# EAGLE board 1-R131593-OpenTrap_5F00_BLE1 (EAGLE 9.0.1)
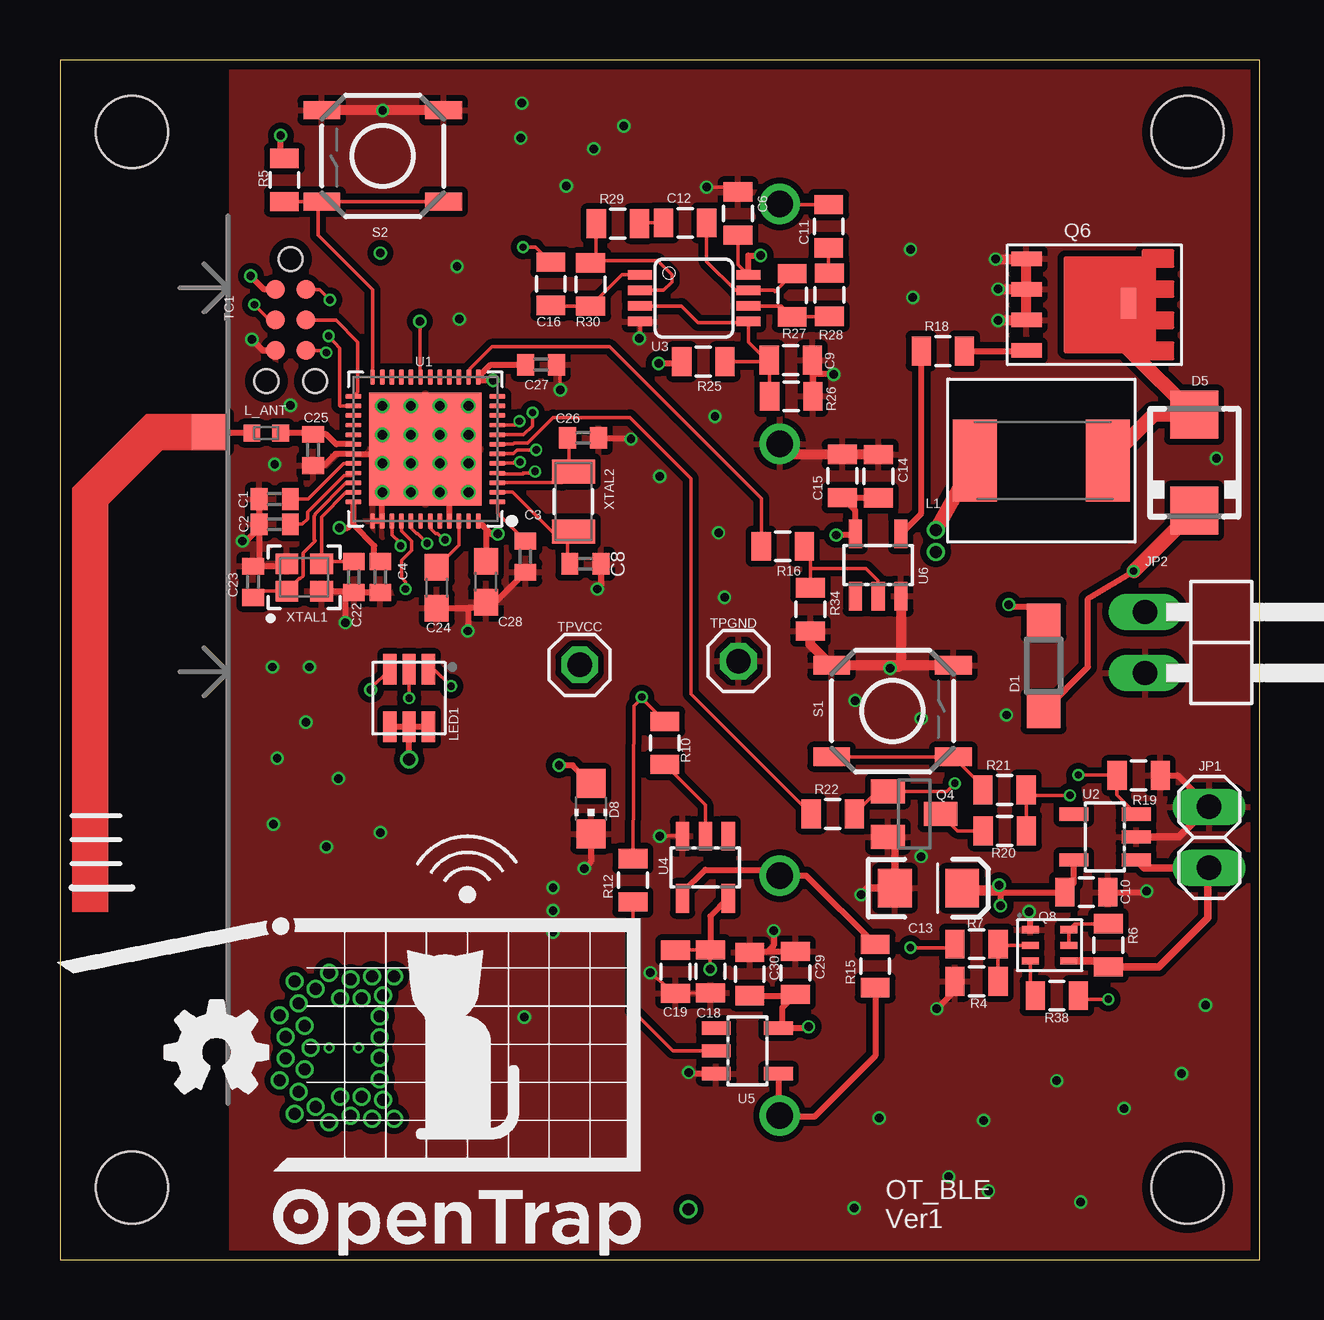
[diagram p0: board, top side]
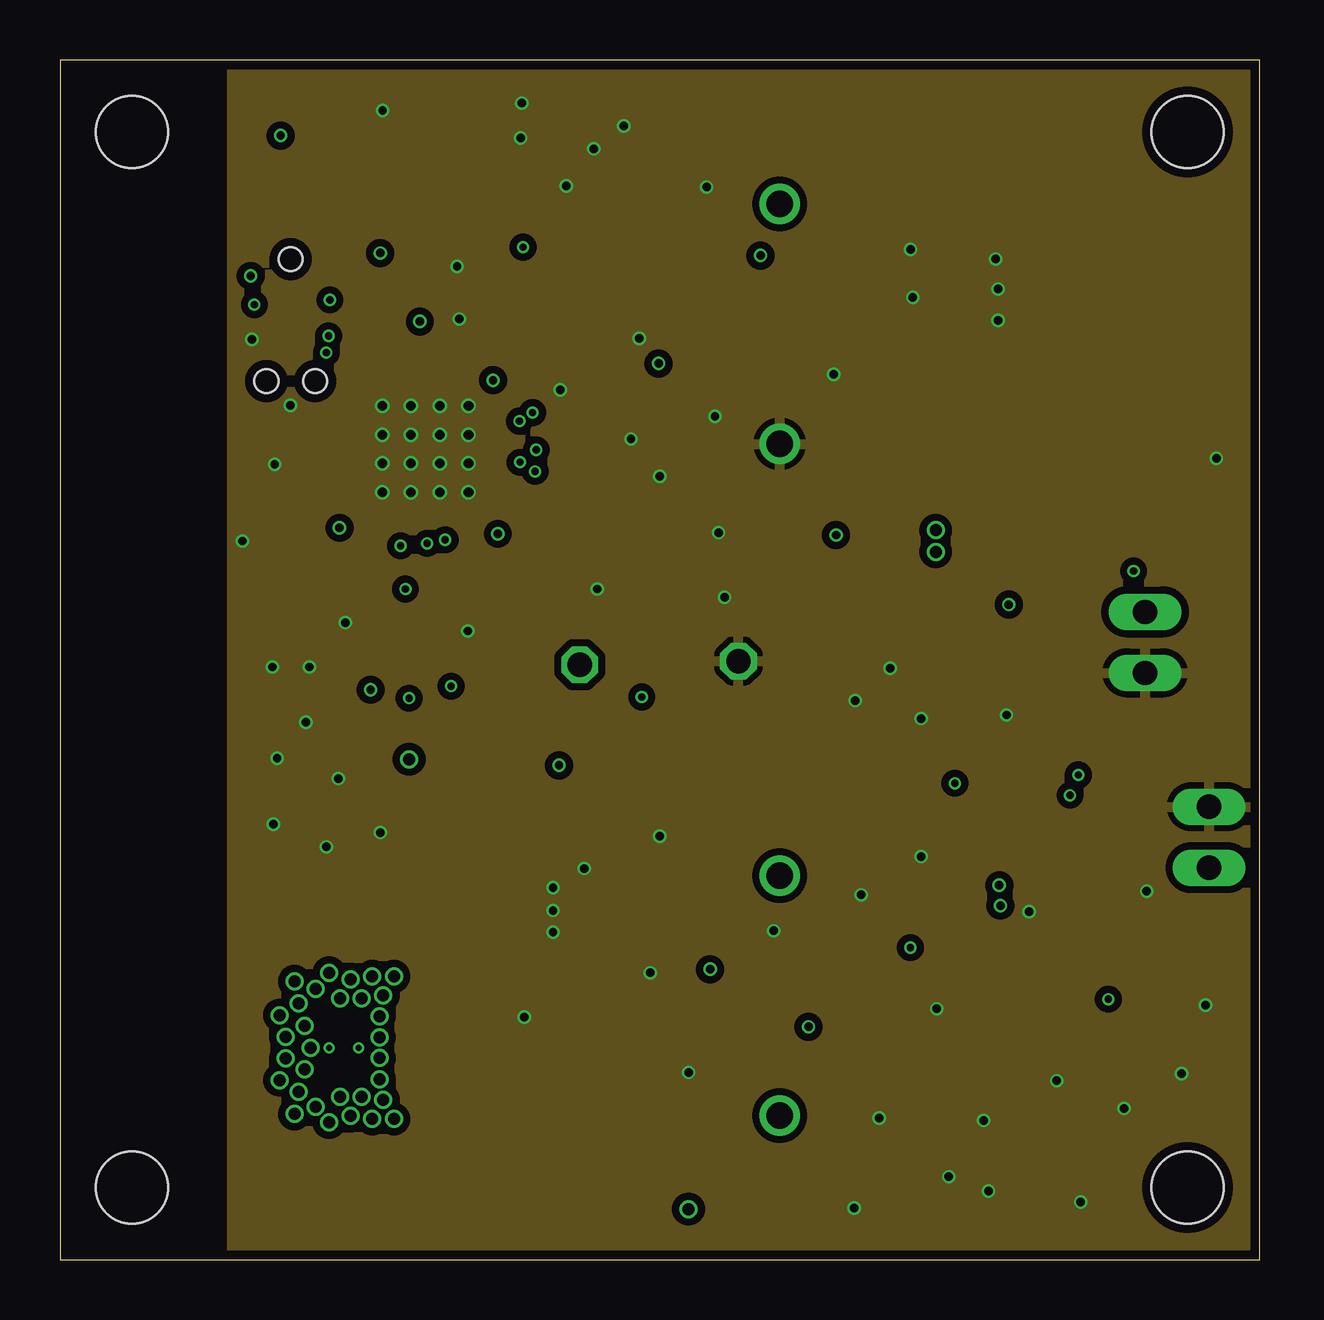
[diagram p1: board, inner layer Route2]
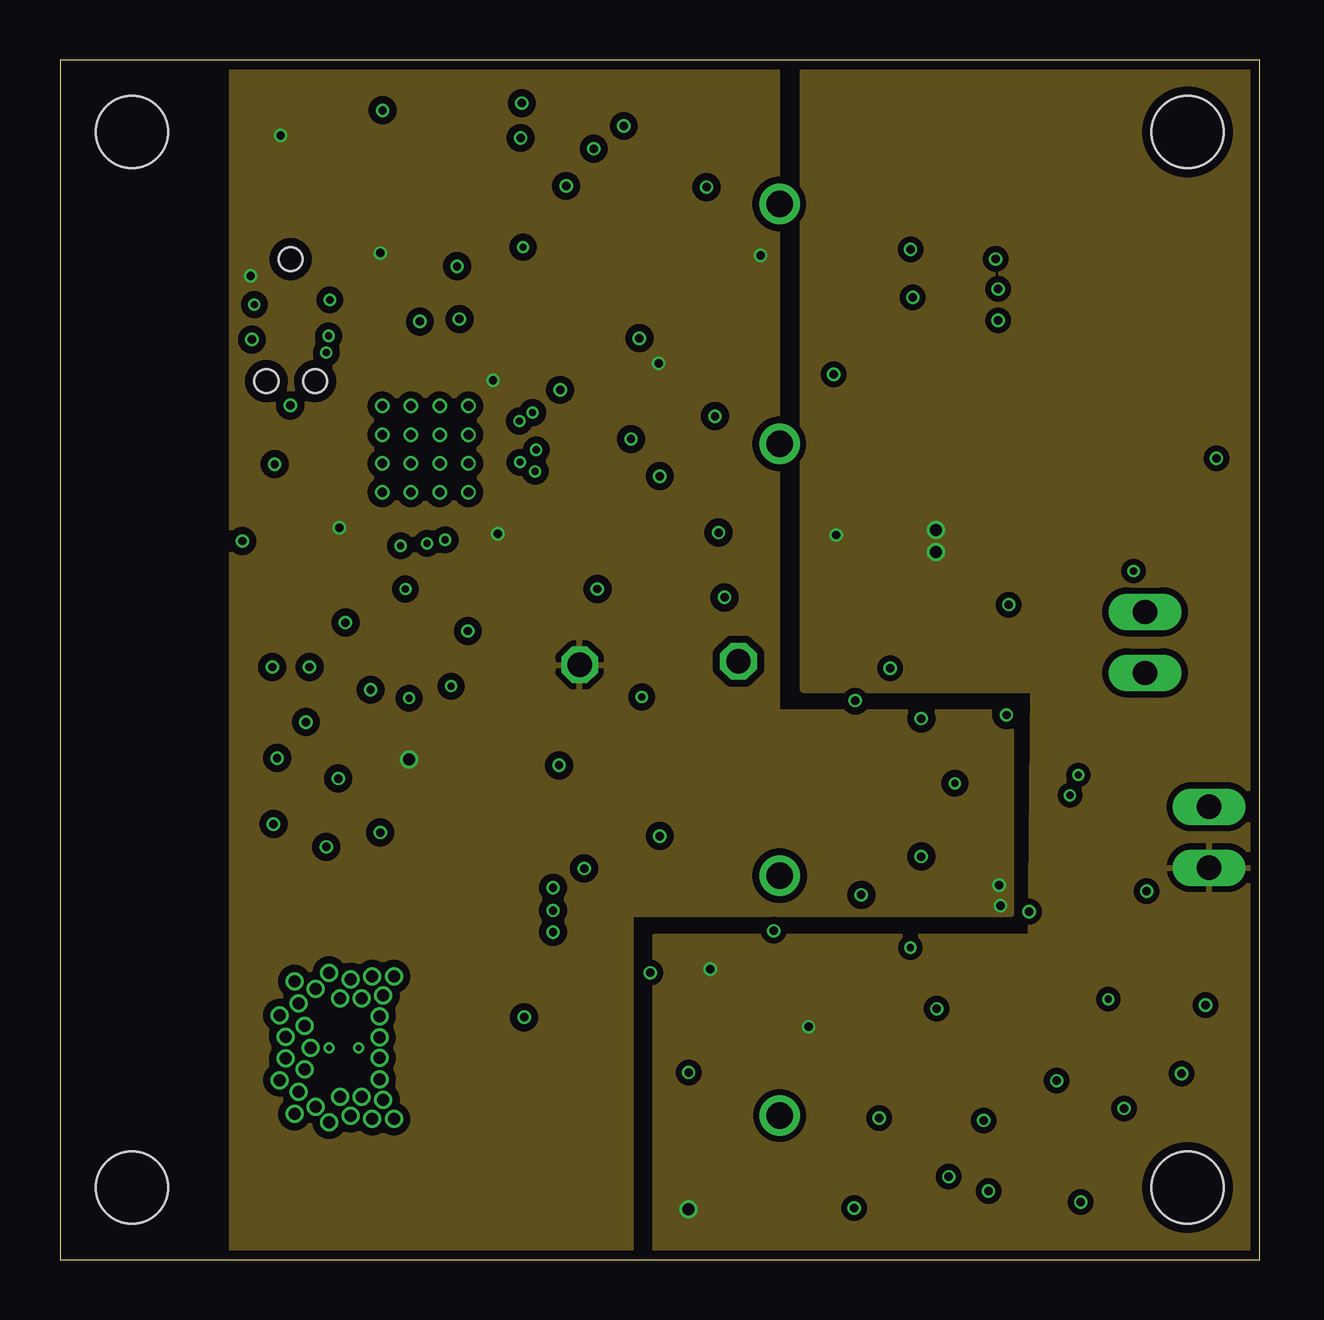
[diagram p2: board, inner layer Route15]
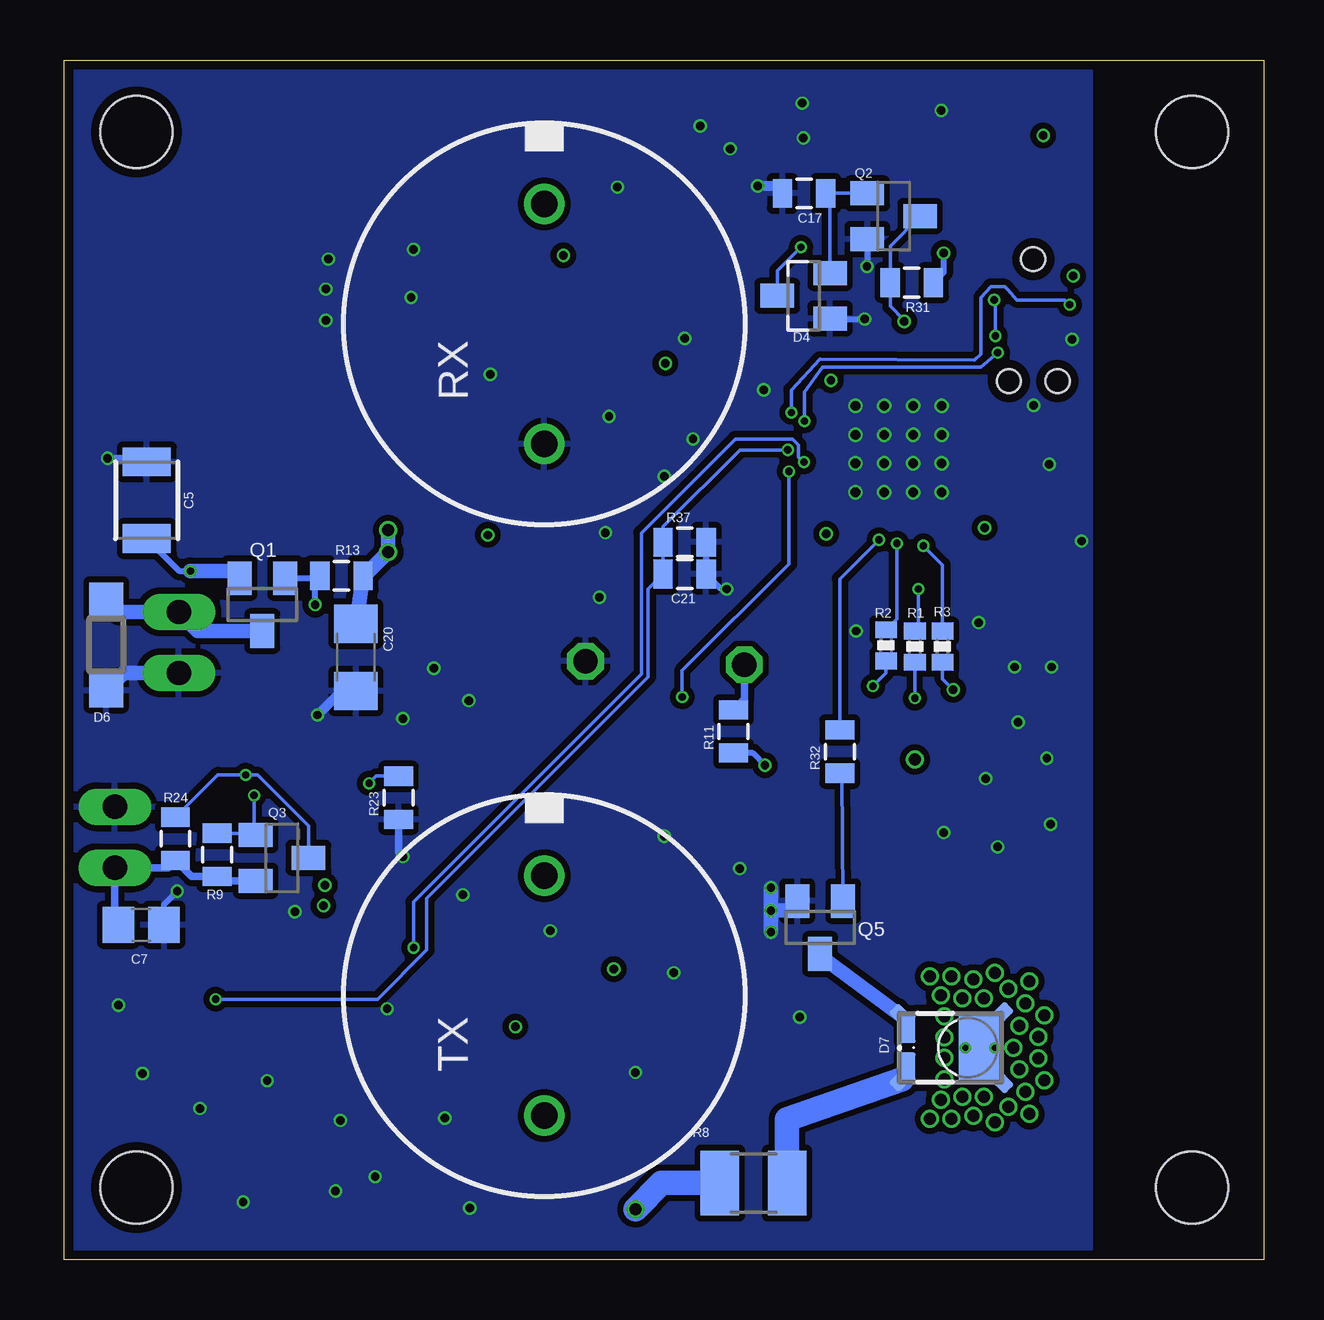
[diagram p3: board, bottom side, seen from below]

Size 50 x 50 mm. Coordinates in mm from the lower left corner, seen from the top.
Outline: 0,0 50,0 50,50 0,50 0,0
Copper layers (1*2*15*16): Top 0.035559375mm / dielectric 0.17018125mm / Route2 0.01778125mm / dielectric 47mil / Route15 0.01778125mm / dielectric 0.17018125mm / Bottom 0.035559375mm
Design rules "oshpark-4layer *": minimum track width 5mil, minimum drill 10mil, track to track 5mil, track to pad 5mil, pad to pad 5mil, via to via 5mil, smd to smd 5mil, copper to edge 15mil, drill to drill 6mil, minimum pad ring 4mil, minimum via ring 4mil, stop-mask expansion 2.5mil, vias tented up to drill 0mil, thermal gap 10mil
Net classes: 1 vcc: width 0.254 mm; 2 GPIO: width 0.152 mm; 3 boost: width 0.381 mm
Holes 3 mm at 3,47 3,3 47,3 47,47

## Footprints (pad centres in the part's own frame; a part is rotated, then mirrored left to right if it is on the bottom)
QWMP_BEND_LEFT_+1 = smd 1.5 x 1.5: P$1 0.75,0
C0402 = smd 0.7 x 0.9: 1 -0.65,0; 2 0.65,0
1210 = smd 1.2 x 2: 1 -1.6,0; 2 1.6,0
0805 = smd 0.8 x 1.2: 1 -0.9,0; 2 0.9,0
C0805 = smd 1.3 x 1.5: 1 -0.95,0; 2 0.95,0
EIA3216 = smd 1.4 x 1.6: A 1.4,0; C -1.4,0
1206 = smd 1.6 x 1.8: 1 -1.4,0; 2 1.4,0
C0603 = smd 1.1 x 1: 1 -0.85,0; 2 0.85,0
SOD123 = smd 1.4 x 1.4: A 1.9,0; C -1.9,0
SOT23 = smd 1 x 1.4: 1 -0.95,-1.1; 2 0.95,-1.1; 3 0,1.1
SMA = smd 2 x 2: A 2,0; C -2,0
LUXEON_REBEL+COOLPAD = smd 1.2 x 0.67: A 0.8,-2.51; C -0.8,-2.51 | smd 1 x 0.6 rotated 315: A@1 1.31,-2.75 | smd 1 x 0.6 rotated 225: C@1 -1.31,-2.75 | smd 2.8 x 1.77: TH 0,0.51 | smd 1 x 0.6 rotated 135: TH@1 -1.39,1.39 | smd 1 x 0.6 rotated 45: TH@2 1.39,1.39 | drill 0.5 pad 0.6: TH@3 2.971,-1.57; TH@4 2.971,-0.67; TH@5 2.85,0.23; TH@6 2.05,0.68; TH@7 2.05,-0.22; TH@8 2.171,-1.12; TH@9 2.764,2.575; TH@10 3.116,1.13; TH@11 2.461,1.687; TH@12 1.844,2.394; TH@13 0.9,2.15; TH@14 0,1.9; TH@15 0.45,2.95; TH@16 1.356,3.196; TH@17 1.31,-0.97; TH@18 0.43,-0.97; TH@21 -2.971,-1.57; TH@22 -2.971,-0.67; TH@23 -2.85,0.23; TH@24 -2.05,0.68; TH@25 -2.05,-0.22; TH@26 -2.171,-1.12; TH@27 -2.764,2.575; TH@28 -3.116,1.13; TH@29 -2.461,1.687; TH@30 -1.844,2.394; TH@31 -0.9,2.15; TH@32 -0.45,2.95; TH@33 -1.356,3.196; TH@34 -1.31,-0.97; TH@35 -0.43,-0.97 | drill 0.25 pad 0.4: TH@19 0,-0.095; TH@20 0,1.125
CHIP-LED0805 = smd 1.2 x 1.2: A 0,-1.05; C 0,1.05
1X02 = drill 1.016 long: 1 -1.27,0; 2 1.27,0
1X02/90 = drill 1.016 long: 1 -1.27,-3.81; 2 1.27,-3.81
ILHM2525 = smd 1.83 x 3.43: 1 -2.77,0; 2 2.77,0
RESC0402_M = smd 0.7 x 0.7: 1 -0.6,0; 2 0.6,0
CLY6D-FKC = smd 0.55 x 1.27: P$1 -0.8,-1.2; P$2 0,-1.2; P$3 0.8,-1.2; P$4 0.8,1.2; P$5 0,1.2; P$6 -0.8,1.2
SOT23-BEC = smd 1 x 1.4: B -0.95,-1.1; C 0,1.1; E 0.95,-1.1
FAIRCHILD56-8 = smd 0.61 x 1.27: 1 -1.91,-2.95; 2 -0.64,-2.95; 3 0.64,-2.95; 4 1.91,-2.95 | smd 1.27 x 0.635: 5-8 -0.05,1.3
SOT363 = smd 0.3 x 0.7: P$1 -0.65,-0.8; P$2 0,-0.8; P$3 0.65,-0.8; P$4 0.65,0.8; P$5 0,0.8; P$6 -0.65,0.8
0402-RES = smd 0.7 x 0.9: 1 -0.65,0; 2 0.65,0
R1210 = smd 1.6 x 2.7: 1 -1.4,0; 2 1.4,0
EFBAA40D101 = drill 1.1 pad 1.676: 1 -5,0; 2 5,0
TACTILE_SWITCH_SMD = smd 1.524 x 0.762: 1 -2.54,1.905; 2 2.54,1.905; 3 -2.54,-1.905; 4 2.54,-1.905
TC2030-IDC-NL = smd 0.787 x 0.787: 1 -1.27,-0.635; 2 -1.27,0.635; 3 0,-0.635; 4 0,0.635; 5 1.27,-0.635; 6 1.27,0.635 | hole 0.991: -2.54,0; 2.54,1.016; 2.54,-1.016
1X01 = drill 1.016 octagon: 1 0,0
QFN40P600X600X90-48_N = smd 0.65 x 0.2: 1 -3,2.2; 2 -3,1.8; 3 -3,1.4; 4 -3,1; 5 -3,0.6; 6 -3,0.2; 7 -3,-0.2; 8 -3,-0.6; 9 -3,-1; 10 -3,-1.4; 11 -3,-1.8; 12 -3,-2.2; 25 3,-2.2; 26 3,-1.8; 27 3,-1.4; 28 3,-1; 29 3,-0.6; 30 3,-0.2; 31 3,0.2; 32 3,0.6; 33 3,1; 34 3,1.4; 35 3,1.8; 36 3,2.2 | smd 0.2 x 0.65: 13 -2.2,-3; 14 -1.8,-3; 15 -1.4,-3; 16 -1,-3; 17 -0.6,-3; 18 -0.2,-3; 19 0.2,-3; 20 0.6,-3; 21 1,-3; 22 1.4,-3; 23 1.8,-3; 24 2.2,-3; 37 2.2,3; 38 1.8,3; 39 1.4,3; 40 1,3; 41 0.6,3; 42 0.2,3; 43 -0.2,3; 44 -0.6,3; 45 -1,3; 46 -1.4,3; 47 -1.8,3; 48 -2.2,3 | smd 4.7 x 4.7: PAD 0,0 | drill 0.4: PAD@VIA01 -1.8,1.8; PAD@VIA02 -1.8,0.6; PAD@VIA03 -1.8,-0.6; PAD@VIA04 -1.8,-1.8; PAD@VIA05 -0.6,1.8; PAD@VIA06 -0.6,0.6; PAD@VIA07 -0.6,-0.6; PAD@VIA08 -0.6,-1.8; PAD@VIA09 0.6,1.8; PAD@VIA10 0.6,0.6; PAD@VIA11 0.6,-0.6; PAD@VIA12 0.6,-1.8; PAD@VIA13 1.8,1.8; PAD@VIA14 1.8,0.6; PAD@VIA15 1.8,-0.6; PAD@VIA16 1.8,-1.8
SOT23-5 = smd 0.55 x 1.2: 1 -0.95,-1.3; 2 0,-1.3; 3 0.95,-1.3; 4 0.95,1.3; 5 -0.95,1.3
MSOP08 = smd 0.4 x 1: 1 -0.976,-2.263; 2 -0.326,-2.263; 3 0.324,-2.263; 4 0.974,-2.263; 5 0.974,2.262; 6 0.324,2.262; 7 -0.326,2.262; 8 -0.976,2.262
SOT23-DBV = smd 0.55 x 1.2: 1 -0.95,-1.3; 2 0,-1.3; 3 0.95,-1.3; 4 0.95,1.3; 5 -0.95,1.3
BT-XTAL_2016_N = smd 0.95 x 0.85: 1 -0.725,-0.575; 2 0.725,-0.575; 3 0.725,0.575; 4 -0.725,0.575
XTAL_3215_N = smd 1 x 1.8: 1 -1.25,0; 2 1.25,0

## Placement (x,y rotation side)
ANT1  ANTENNA_QUARTER-WAVE_MONOPOLE_BEND_LEFT+1  [QWMP_BEND_LEFT_+1]  7,34.5 180 top
C1  DNI  [C0402]  8.95,31.7 180 top
C2  100PF  [C0402]  8.95,30.65 180 top
C3  .1u  [C0402]  19.4,29.3 270 top
C4  0.1uF  [C0402]  13.35,28.45 270 top
C5  22uF  [1210]  46.57,31.65 270 bottom
C6  0.1uF  [0805]  28.26,43.6 270 top
C7  22uF  [C0805]  46.8,13.95 0 bottom
C8  12pF  [C0402]  21.9,29 180 top
C9  0.1uF  [0805]  30.46,37.49 180 top
C10  0.1uF  [0805]  42.78,15.31 0 top
C11  1000pF  [0805]  32.04,43.07 90 top
C12  1000pF  [0805]  26.06,43.21 0 top
C13  10uF  [EIA3216]  36.2,15.48 0 top
C14  1uF  [0805]  34.11,32.65 270 top
C15  0.1uF  [0805]  32.61,32.66 270 top
C16  1  [0805]  20.46,40.67 270 top
C17  .1uF  [0805]  19.17,44.44 180 bottom
C18  1uF  [0805]  27.11,12.01 90 top
C19  0.1uF  [0805]  25.66,12 90 top
C20  22uF  [1206]  37.85,25.1 270 bottom
C21  .1uF  [0805]  24.15,28.57 0 bottom
C22  12pF  [C0402]  12.25,28.45 270 top
C23  12pF  [C0402]  8.05,28.25 90 top
C24  1uF  [C0603]  15.7,28 270 top
C25  .8pF  [C0402]  10.55,33.75 270 top
C26  12pF  [C0402]  21.8,34.25 180 top
C27  .1uF  [C0402]  20.05,37.3 180 top
C28  4.7uF  [C0603]  17.75,28.25 270 top
C29  1uF  [0805]  30.65,11.95 270 top
C30  0.1uF  [0805]  28.75,11.9 270 top
D1  10V_ZNR_SOD123  [SOD123]  41,24.75 90 top
D4  BAV199  [SOT23]  19.19,40.17 90 bottom
D5  MBRA340T3  [SMA]  47.28,33.21 90 top
D6  [SOD123]  48.26,25.62 270 bottom
D7  LUXEON_REBEL+COOLPAD  [LUXEON_REBEL+COOLPAD]  12.35,8.83 270 bottom
D8  [CHIP-LED0805]  22.13,18.79 180 top
JP1  [1X02]  47.9,17.6 90 top
JP2  [1X02/90]  49.04,25.72 270 top
L1  4.7uH  [ILHM2525]  40.91,33.3 0 top
L_ANT  3.9nH  [RESC0402_M]  8.6,34.45 180 top
LED1  CLY6D-FKC  [CLY6D-FKC]  14.55,23.4 180 top
Q1  DMP1045UQ  [SOT23]  41.75,27.3 180 bottom
Q2  [SOT23-BEC]  15.44,43.49 270 bottom
Q3  MMBT2907ALT1SMD  [SOT23-BEC]  40.93,16.74 270 bottom
Q4  [SOT23]  35.61,18.57 270 top
Q5  [SOT23]  18.5,13.84 180 bottom
Q6  FC56-8  [FAIRCHILD56-8]  43.24,39.8 270 top
Q8  BSD235C  [SOT363]  41.25,13.1 270 top
R1  1K  [0402-RES]  14.55,25.55 270 bottom
R2  1K  [0402-RES]  15.75,25.6 270 bottom
R3  1K  [0402-RES]  13.4,25.55 270 bottom
R4  220K  [0805]  38.2,11.6 0 top
R5  10k  [0805]  9.35,45 270 top
R6  10K  [0805]  43.7,13.1 270 top
R7  1K  [0805]  38.2,13.15 180 top
R8  15ohm  [R1210]  21.28,3.19 0 bottom
R9  47K  [0805]  43.64,16.87 270 bottom
R10  1K  [0805]  25.21,21.53 90 top
R11  1K  [0805]  22.11,22.01 90 bottom
R12  1K  [0805]  23.88,15.81 90 top
R13  10K  [0805]  38.45,28.5 180 bottom
R15  1M  [0805]  33.98,12.23 90 top
R16  1K  [0805]  30.13,29.73 180 top
R18  1K  [0805]  36.8,37.87 0 top
R19  220K  [0805]  44.96,20.18 180 top
R20  10K  [0805]  39.38,17.87 0 top
R21  10K  [0805]  39.37,19.57 0 top
R22  1K  [0805]  32.21,18.57 0 top
R23  220K  [0805]  36.07,19.25 90 bottom
R24  DNI  [0805]  45.37,17.54 90 bottom
R25  7.87k  [0805]  26.82,37.43 180 top
R26  7.87k  [0805]  30.48,35.98 180 top
R27  33k  [0805]  30.52,40.19 270 top
R28  4.99k  [0805]  32.07,40.21 90 top
R29  4.99k  [0805]  23.25,43.18 0 top
R30  100k  [0805]  22.12,40.64 90 top
R31  1K  [0805]  14.68,40.72 180 bottom
R32  1K  [0805]  17.68,21.17 90 bottom
R34  10K  [0805]  31.28,27.1 270 top
R37  1.21K  [0805]  24.15,29.9 0 bottom
R38  9.2K  [0805]  41.55,11 0 top
RX  EFBAA40D101  [EFBAA40D101]  30,39 90 bottom
S1  Poweron  [TACTILE_SWITCH_SMD]  34.7,22.86 0 top
S2  reset  [TACTILE_SWITCH_SMD]  13.45,46 180 top
TC1  TC2030-IDC-NL  [TC2030-IDC-NL]  9.62,39.16 270 top
TPGND  [1X01]  28.28,24.94 0 top
TPVCC  [1X01]  21.66,24.79 0 top
TX  EFBAA40D101  [EFBAA40D101]  30,11 90 bottom
U1  NRF52832  [QFN40P600X600X90-48_N]  15.23,33.78 180 top
U2  MIC5219BM5  [SOT23-5]  43.56,17.61 90 top
U3  MCP6002  [MSOP08]  26.43,40.07 270 top
U4  SN74LV1T34  [SOT23-DBV]  26.9,16.35 180 top
U5  SN74LV1T04  [SOT23-DBV]  28.65,8.7 270 top
U6  SN74LV1T34  [SOT23-DBV]  34.1,28.95 0 top
U$1  [OTLOGO]  -0.35,-0.15 0 top
XTAL1  FA-128 32.0000MF10Z-AJ3  [BT-XTAL_2016_N]  10.18,28.43 0 top
XTAL2  ECS-.327-9-34B-C-TR  [XTAL_3215_N]  21.4,31.6 270 top

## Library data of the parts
ANT1 = Nordic_misc
C1 C4 C24 C27 C28 = rcl; SPICEPREFIX: C
C2 C8 C23 C25 C26 = rcl; DIEL: C0G; SPICEPREFIX: C
C3 = rcl; DIEL: x7r; SPICEPREFIX: C
C5 C6 C9-C21 C29 C30 R1-R7 R9-R13 R15 R16 R18-R32 R34 R37 R38 S1 S2 = SparkFun
C7 R8 = rcl
C22 = rcl; DIEL: c0g; SPICEPREFIX: C
D1 LED1 Q8 U4-U6 U$1 = Roger_lib
D4-D6 = diode
D7 = led-lumiled; OC_FARNELL: unknown; OC_NEWARK: unknown
D8 = led
JP1 JP2 TPGND TPVCC = pinhead
L1 = Rogerlib
L_ANT U1 XTAL1 XTAL2 = Nordic_nRF
Q1 = transistor-small-signal
Q2 = transistor-neu-to92
Q3 = transistor-pnp
Q4 Q5 = adafruit
Q6 = testlibFC56-8
RX TX = buzzer; OC_FARNELL: unknown; OC_NEWARK: unknown
TC1 = TagConnect
U2 = v-reg-micrel; MF: ALTERA CORPORATION; MPN: MIC5219BM5 TR; OC_FARNELL: 1100656; OC_NEWARK: 09J8939
U3 = analog-devices; MPN: AD8656ARMZ; OC_FARNELL: 1117887; OC_NEWARK: 34P3252

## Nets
3.3V [vcc]: C4.1 C6.2 C10.1 C13.A C27.2 C28.1 LED1.P$4 LED1.P$5 LED1.P$6 R5.1 R11.2 R25.2 R31.1 TC1.1 TPVCC.1 U1.13 U1.36 U1.48 U2.5 U3.8
BATT_DIV [GPIO]: C21.1 R37.1 R38.2 U1.6
BST_DRV: R16.2 U1.14
DIV_EN [GPIO]: R7.2 U1.5
EN_PLDN [GPIO]: Q3.B R9.1 R20.2 R21.2
GND [vcc]: C1.2 C2.2 C3.2 C4.2 C5.1 C6.1 C7.2 C8.1 C9.1 C10.2 C13.C C14.1 C15.1 C17.2 C18.1 C19.1 C20.2 C21.2 C22.2 C23.2 C24.2 C25.2 C26.1 C27.1 C28.2 C29.1 C30.1 D4.1 D6.A D8.C JP1.2 JP2.2 Q2.E Q4.2 Q5.2 Q6.1 Q6.2 Q6.3 Q8.P$1 R4.1 R19.1 R23.1 R26.1 R34.2 R37.2 RX.1 S1.1 S1.2 S2.3 S2.4 TC1.5 TPGND.1 U1.31 U1.37 U1.38 U1.45 U1.PAD U1.PAD@VIA01 U1.PAD@VIA02 U1.PAD@VIA03 U1.PAD@VIA04 U1.PAD@VIA05 U1.PAD@VIA06 U1.PAD@VIA07 U1.PAD@VIA08 U1.PAD@VIA09 U1.PAD@VIA10 U1.PAD@VIA11 U1.PAD@VIA12 U1.PAD@VIA13 U1.PAD@VIA14 U1.PAD@VIA15 U1.PAD@VIA16 U2.2 U3.4 U4.3 U5.3 U6.3 XTAL1.2 XTAL1.4
LDO_EN [GPIO]: Q3.C R19.2 R24.2 U2.3
LIGHT: R32.2 U1.43
N$1 [GPIO]: C22.1 U1.35 XTAL1.3
N$2 [GPIO]: C23.1 U1.34 XTAL1.1
N$3 [GPIO]: R18.1 U6.4
N$4 [GPIO]: C1.1 U1.32
N$5 [GPIO]: C2.1 U1.33
N$6 [GPIO]: R16.1 R34.1 U6.2
N$7 [GPIO]: C8.2 U1.2 XTAL2.2
N$8: Q6.4 R18.2
N$9 [GPIO]: C3.1 U1.1
N$10 [GPIO]: C26.2 U1.3 XTAL2.1
N$11 [GPIO]: Q8.P$5 Q8.P$6 R6.1
N$12 [GPIO]: R15.1 TX.1 U5.4
N$13 [GPIO]: R5.2 S2.1 S2.2 U1.24
N$14 [GPIO]: R15.2 TX.2 U4.4
N$15: R3.1 U1.39
N$16: C11.2 RX.2
N$17 [GPIO]: C9.2 R25.1 R26.2 U3.3 U3.5
N$18: C11.1 R28.2
N$19 [GPIO]: R12.1 U5.2
N$20: D7.C D7.C@1 Q5.3
N$21: C12.1 R29.2
N$22: Q5.1 R32.1
N$23: R1.1 U1.40
N$24 [boost]: D7.A D7.A@1 R8.2
N$25: R2.1 U1.41
N$26: LED1.P$3 R3.2
N$27: R21.1 S1.3 S1.4
N$28 [GPIO]: R27.2 R28.1 U3.6
N$29: Q4.3 R20.1
N$30: LED1.P$2 R1.2
N$31 [GPIO]: C12.2 R27.1 U3.7
N$32 [GPIO]: Q4.1 R22.2 R23.2
N$33 [GPIO]: C16.2 R30.1 U3.1
N$34 [GPIO]: R29.1 R30.2 U3.2
N$35 [GPIO]: D6.C JP2.1 Q1.3
N$36: C16.1 D4.3
N$37: LED1.P$1 R2.2
N$38: D8.A R11.1
N$39 [GPIO]: R10.1 U4.2
N$41 [GPIO]: C17.1 D4.2 Q2.B
N$42 [GPIO]: C5.2 D1.C D5.C Q1.2
N$43: C24.1 U1.46
N$44 [boost]: D5.A L1.2 Q6.5-8
N$45 [GPIO]: D1.A Q1.1 R13.2
N$49 [vcc]: C25.1 L_ANT.1 U1.30
N$50 [vcc]: ANT1.P$1 L_ANT.2
N$51: Q8.P$2 R4.2 R7.1
N$53: Q8.P$3 R38.1
P0_06 [GPIO]: TC1.3 U1.8
P0_07 [GPIO]: TC1.6 U1.9
POW_ON [GPIO]: R22.1 U1.7
RCVR_IN: Q2.C R31.2 U1.19
SWDCLK [GPIO]: TC1.4 U1.25
SWDIO [GPIO]: TC1.2 U1.26
TH: D7.TH D7.TH@1 D7.TH@2 D7.TH@3 D7.TH@4 D7.TH@5 D7.TH@6 D7.TH@7 D7.TH@8 D7.TH@9 D7.TH@10 D7.TH@11 D7.TH@12 D7.TH@13 D7.TH@14 D7.TH@15 D7.TH@16 D7.TH@17 D7.TH@18 D7.TH@19 D7.TH@20 D7.TH@21 D7.TH@22 D7.TH@23 D7.TH@24 D7.TH@25 D7.TH@26 D7.TH@27 D7.TH@28 D7.TH@29 D7.TH@30 D7.TH@31 D7.TH@32 D7.TH@33 D7.TH@34 D7.TH@35
VIN [boost]: C7.1 C14.2 C15.2 C18.2 C19.2 C20.1 C29.2 C30.2 JP1.1 L1.1 Q3.E Q8.P$4 R6.2 R8.1 R9.2 R13.1 R24.1 U2.1 U4.5 U5.5 U6.5
XMIT_DRV [GPIO]: R10.2 R12.2 U1.4

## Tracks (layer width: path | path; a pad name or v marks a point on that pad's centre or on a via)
3.3V  (via drill 0.35, 0.5)
  Top 0.152: U3.8 28.26,41.48 C6.2
  Top 0.254: C27.2 17.95,37.3 U1.13 17.56,36.65 v18.05,36.65 | C28.1 17.75,30.46 U1.48 17.96,30.25 v18.25,30.25 | C4.1 13.1,29.35 13.1,29.75 12.23,30.62 12.23,30.75 | 12.23,30.75 U1.36 | U2.5 42.26,15.69 C10.1 37.77,15.31 C13.A 39.03,15.48 v39.15,15.6 39.2,15.55 v39.2,14.75 | LED1.P$6 LED1.P$5 | LED1.P$5 LED1.P$4 | v14.55,20.85 LED1.P$5 | R5.1 9.2,45.9 v9.2,46.85 | U3.8 28.69,41.85 v29.2,41.85 | TC1.1 8.52,40.43 v7.95,41 | R25.2 25.84,37.35 v24.95,37.35 | v11.65,30.5 11.98,30.5 12.23,30.75
  Bottom 0.254: R31.1 13.35,41.15 v13.35,41.95
  Bottom 0.305: R11.2 21.66,23.36 TPVCC.1
  pour Route15 (isolate 0.305): 7.15,52.15 7.15,-0.85 23.8,-0.85 23.8,14.4 39.65,14.4 39.65,22.8 29.9,22.8 29.9,52.15
BATT_DIV  (via drill 0.3)
  Top 0.152: U1.6 arc-90 18.25,33.6 18.9,33.6 19.05,33.75 v19.85,33.75 | v43.7,10.85 42.6,10.85 R38.2
  Bottom 0.152: v19.85,33.75 21.85,33.75 25.05,30.55 R37.1 C21.1 25.67,27.95 25.67,24.28 34.9,15.05 34.9,12.91 36.96,10.85 v43.7,10.85 43.75,10.85
BST_DRV
  Top 0.152: R16.2 29.23,31.72 22.9,38.05 18,38.05 17.1,37.15 17.1,36.85 U1.14
DIV_EN  (via drill 0.3)
  Top 0.152: U1.5 arc-90 18.25,33.2 18.9,33.2 18.93,33.23 v19.18,33.23 | v35.45,13 37.15,13 R7.2
  Bottom 0.152: v19.18,33.23 19.39,33.45 19.39,33.94 19.66,34.2 22.03,34.2 25.95,30.29 25.95,24.4 35.45,14.9 v35.45,13
EN_PLDN  (via drill 0.3)
  Top 0.152: R20.2 R21.2 | R21.2 | v42.1,19.35 40.49,19.35 R21.2
  Bottom 0.152: R9.1 42.11,17.77 Q3.B 42.1,17.76 v42.1,19.35
GND  (via drill 0.35)
  Top 0.152: C27.1 20.85,37.3 v20.85,36.25 | U3.4 24.17,38.4 v24.15,38.4 | C6.1 arc90 28.06,44.7 v26.95,44.7 | U4.3 v25,17.65 | C18.1 C19.1 v24.6,11.95
  Top 0.254: C25.2 11,33.1 11.48,33.58 U1.31 13.97,33.58 14.05,33.5 13.73,33.18 U1.PAD@VIA14 | U1.38 13.4,30.78 | 13.4,30.78 U1.37 | U1.PAD 13.4,31.95 13.4,30.78 | U1.45 16.23,31.47 15.83,31.87 U1.PAD@VIA05 | 15.23,34.38 U1.PAD@VIA15 | U1.PAD 15.23,34.38 | 15.23,34.38 U1.PAD@VIA03 | U1.PAD 15.83,33.78 U1.PAD@VIA06 | C9.1 31.38,37.49 31.38,36.9 | 31.38,36.9 R26.1 | v32.25,36.9 31.38,36.9 | XTAL1.4 9.46,28.9 C23.2 8.3,29.15 8.3,30.5 | XTAL1.2 12.25,27.86 C22.2 | C4.2 C22.2 | v11.9,26.55 11.9,27.8 C22.2 | C24.2 17,27.15 | 17,27.15 v17,26.2 | 17,27.15 17.75,27.15 C28.2 18.15,27.4 C3.2 | C1.2 C2.2 8.3,30.5 | v7.6,29.95 7.75,29.95 8.3,30.5 | D8.C 22.13,16.58 v21.85,16.3 | U5.3 26.25,7.75 v26.2,7.8 | C30.1 28.8,12.85 29.5,12.85 | 29.5,12.85 C29.1 | v29.75,13.7 29.75,13.1 29.5,12.85 | C10.2 45.26,15.31 v45.3,15.35 | R4.1 37.3,11.2 v36.55,10.45 | TC1.5 8.46,37.89 v8,38.35 | C8.1 22.55,28.1 v22.4,27.95 | C26.1 23.75,34.25 v23.8,34.2 | Q8.P$1 40.45,14.45 v40.4,14.5 | R19.1 46.59,20.18 JP1.2
  Top 0.305: U2.2 46.64,17.61 JP1.2 | v34.6,24.65 34.98,24.65 35.1,24.77 | v33.4,15.2 33.68,15.48 C13.C 34.8,17.33 Q4.2
  Top 0.406: Q6.2 Q6.3 v39.1,39.15 | Q6.2 Q6.1 v39,41.7 | v39.1,40.45 Q6.2 | C14.1 C15.1 30.44,33.56 RX.1 | S1.2 35.1,24.77 | 35.1,24.77 S1.1 31.28,25.64 R34.2 | U6.3 35.05,24.82 35.1,24.77 | S2.4 S2.3 v13.45,47.9
  Bottom 0.254: D4.1 18.09,39.2 v16.65,39.2 | Q2.E v16.54,41.4 v16.55,41.4 | C5.1 arc-90 46.72,33.4 v48.2,33.4 | C7.2 45.85,14.8 v45.3,15.35 | R37.2 C21.2 22.62,27.95 v22.4,27.95
  Bottom 0.305: R23.1 36.07,16.97 v35.9,16.8
  Bottom 0.406: C20.2 38.45,23.7 v39.45,22.7 | C17.2 20.07,44.75 v21.1,44.75
  Bottom 0.61: JP2.2 47.53,24.45 D6.A | v20.55,13.65 v20.55,14.55 | v20.55,14.55 v20.55,15.5 | Q5.2 19.84,14.55 v20.55,14.55
  other vias: 33.15,23.3 35.9,22.55 8.85,24.7 10.4,24.7 8.95,33.15 11.6,20.05 9.05,20.9 8.9,18.15 10.25,22.4 13.35,17.8 11.1,17.2 9.6,35.6 19.35,10.1 38.7,2.85 33.1,2.15 34.15,5.9 44.35,6.3 41.55,7.45 38.5,5.8 37.05,3.45 42.55,2.4 46.75,7.75 47.75,10.6 35.55,40.1 35.45,42.1 22.25,46.3 23.5,47.25 19.25,48.2 19.2,46.75 27.7,27.6 27.45,30.3 25,32.65 27.3,35.15
  pour Route2 (isolate 0.305): 7.15,43.55 7.15,-2.1 7.75,-2.1 51.45,-2.1 51.45,0.65 51.45,50.95 49.75,50.95 7.15,50.95
  pour Bottom (isolate 0.254): 7.25,51.45 7.25,-0.8 51.8,-0.8 51.8,51.5 7.25,51.5
  pour Top (isolate 0.254): 7.15,53.5 7.15,-0.7 9.85,-0.7 50.85,-0.7 50.85,6.45 50.85,53.5
LDO_EN  (via drill 0.3)
  Top 0.152: v42.45,20.2 44.04,20.2 R19.2 44.06,19.36 U2.3
  Bottom 0.152: Q3.C 39.83,18.08 41.95,20.2 v42.45,20.2 43.61,20.2 R24.2
LIGHT  (via drill 0.3)
  Top 0.152: U1.43 15.43,30.48 15.66,30.25 15.75,30.25 16,30 v16.05,30
  Bottom 0.152: v16.05,30 17.68,28.37 R32.2
N$1
  Top 0.152: U1.35 12.21,31.96 11.91,31.96 10.9,30.95 10.9,29.1 | 10.9,29.1 XTAL1.3 | C22.1 10.9,29.1
N$2
  Top 0.152: U1.34 11.94,32.38 10.63,31.07 10.63,31.03 10.6,31 10.6,30 10.63,29.97 10.63,29.95 10.13,29.46 10.13,28.5 10.01,28.38 9.98,28.38 XTAL1.1 8.3,27.86 C23.1
N$3
  Top 0.254: U6.4 35.9,31.1 R18.1
N$4
  Top 0.152: U1.32 11.83,33.18 10.35,31.7 C1.1
N$5
  Top 0.152: C2.1 10.1,30.65 10.32,30.87 10.32,31.16 11.84,32.68 12.13,32.68 U1.33
N$6
  Top 0.152: R34.1 31.28,28.8 | 31.28,28.8 31.28,29.48 R16.1 | U6.2 34.1,28.3 33.6,28.8 31.28,28.8
N$7
  Top 0.152: XTAL2.2 21.15,30.35 | 21.15,30.35 20.5,30.35 18.87,31.98 U1.2 | C8.2 21.15,29.1 21.15,30.35
N$8
  Top 0.254: R18.2 40.27,37.87 Q6.4
N$9
  Top 0.152: C3.1 18.23,31.12 U1.1
N$10
  Top 0.152: XTAL2.1 21.23,32.67 | 21.23,32.67 20.93,32.38 U1.3 | C26.2 21.23,34.17 21.23,32.67
N$11
  Top 0.152: R6.1 42.3,14 Q8.P$6 Q8.P$5
N$12
  Top 0.254: 30.1,5.95 31.45,5.95 33.98,8.48 R15.1 33.94,11.29 | 30.1,5.95 30.05,5.95 TX.1 | U5.4 29.95,6.1 30.1,5.95
N$13
  Top 0.152: S2.1 10.95,44.09 | 10.95,44.09 S2.2 R5.2 | U1.24 13.03,40.42 10.75,42.7 10.75,43.9 10.95,44.09
N$14
  Top 0.254: R15.2 31.11,16 TX.2 29.75,16.25 26.9,16.25 25.95,15.3 U4.4
N$15  (via drill 0.3)
  Top 0.152: U1.39 13.85,30.76 13.85,30.2 14.15,29.9 14.2,29.9 v14.2,29.75
  Bottom 0.152: v14.2,29.75 13.4,28.95 R3.1
N$16
  Top 0.152: C11.2 30.03,43.97 RX.2
N$17
  Top 0.152: U3.3 25.9,39.75 26.6,39.05 28.65,39.05 U3.5 28.69,38.24 29.5,37.43 | R25.1 29.5,37.43 | 29.5,37.43 C9.2 | R26.2 29.58,37.35 29.5,37.43
N$18
  Top 0.152: C11.1 32.04,41.14 R28.2
N$19
  Top 0.152: U5.2 25.55,8.7 23.88,10.37 R12.1
N$20
  Bottom 0.61: D7.C@1 18.55,12.69 Q5.3
N$21
  Top 0.152: C12.1 24.18,43.21 R29.2
N$22
  Bottom 0.152: R32.1 17.6,20.19 Q5.1
N$23  (via drill 0.3)
  Top 0.152: U1.40 14.23,30.36 14.65,29.94 14.65,29.56 14.23,29.14 14.23,28.42 14.4,28.25 v14.4,27.95
  Bottom 0.152: v14.4,27.95 14.4,26.35 R1.1
N$24
  Bottom 1.016: R8.2 19.88,5.84 D7.A@1
N$25  (via drill 0.3)
  Top 0.152: v15.3,29.85 14.9,30.25 14.86,30.25 14.63,30.48 U1.41
  Bottom 0.152: R2.1 15.3,26.7 v15.3,29.85
N$26  (via drill 0.35)
  Top 0.152: LED1.P$3 12.95,23.8 v12.95,23.75 12.95,23.7
  Bottom 0.152: v12.95,23.75 13.4,24.2 R3.2
N$27
  Top 0.152: R21.1 38.47,19.73 S1.4 S1.3
N$28
  Top 0.152: R28.1 30.54,39.31 R27.2 30.06,39.75 U3.6
N$29
  Top 0.152: Q4.3 37.41,17.87 R20.1
N$30  (via drill 0.3)
  Top 0.152: LED1.P$2 v14.55,23.4
  Bottom 0.152: v14.55,23.4 R1.2
N$31
  Top 0.152: R27.1 30.52,41.07 29.8,40.35 29.75,40.4 U3.7 28.15,40.4 26.95,41.6 C12.2
N$32  (via drill 0.3)
  Top 0.152: R22.2 34.06,19.52 Q4.1 36.97,19.52 v37.3,19.85
  Bottom 0.152: v37.3,19.85 37,20.15 R23.2
N$33
  Top 0.152: U3.1 23.43,41.05 R30.1 20.49,39.74 C16.2
N$34
  Top 0.152: R29.1 22.35,41.77 22.21,41.63 | 22.21,41.63 R30.2 | U3.2 25.15,40.4 25.5,40.75 25.5,41.05 24.91,41.63 22.21,41.63
N$35
  Bottom 0.61: Q1.3 44.44,26.2 JP2.1 47.73,26.99 D6.C
N$36  (via drill 0.3)
  Top 0.152: C16.1 19.83,42.2 v19.3,42.2
  Bottom 0.152: D4.3 20.29,41.21 v19.3,42.2
N$37  (via drill 0.3)
  Top 0.152: LED1.P$1 15.6,24.6 v16.3,23.9
  Bottom 0.152: R2.2 15.75,24.45 v16.3,23.9
N$38  (via drill 0.35)
  Top 0.254: D8.A 21.37,20.6 v20.8,20.6
  Bottom 0.254: v20.8,20.6 21.31,21.11 R11.1
N$39
  Top 0.152: R10.1 26.9,18.94 U4.2
N$41
  Bottom 0.152: D4.2 18.09,44.26 C17.1 Q2.B
N$42  (via drill 0.3)
  Top 0.254: D1.C 42.85,24.7 42.85,27.55 v44.75,28.7
  Top 0.61: D5.C 44.77,28.7 v44.75,28.7
  Bottom 0.254: C5.2 45.22,28.7 v44.75,28.7
  Bottom 0.61: v44.75,28.7 43,28.7 Q1.2
N$43
  Top 0.152: U1.46 16.63,29.78 C24.1
N$44
  Top 0.61: Q6.5-8 44.54,37.95 D5.A 45.59,35.21 L1.2
N$45  (via drill 0.35)
  Top 0.254: D1.A 40.45,27.2 39.5,27.2 39.55,27.25 v39.55,27.3
  Bottom 0.254: v39.55,27.3 39.55,28.3 R13.2 39.45,28.4 Q1.1
N$49
  Top 0.254: U1.30 11.52,33.98 11.1,34.4 C25.1 10.5,34.45 L_ANT.1
N$50
  Top 0.254: ANT1.P$1 6.3,34.45 L_ANT.2
N$51
  Top 0.152: R4.2 39.1,13.1 | 39.1,13.1 R7.1 | Q8.P$2 39.1,13.1
N$53
  Top 0.152: R38.1 40.45,11.2 Q8.P$3
P0_06  (via drill 0.3)
  Top 0.152: TC1.3 8.74,39.16 v8.1,39.8 | U1.8 19.33,34.38 19.7,34.75 v19.7,35.3
  Bottom 0.152: v8.1,39.8 8.3,40 10.3,40 10.68,40.42 10.8,40.55 10.95,40.55 11.39,40.55 11.8,40.09 11.8,37.75 12.07,37.48 18.52,37.53 19.7,36.24 v19.7,35.3
P0_07  (via drill 0.3)
  Top 0.152: TC1.6 10.96,37.89 11.05,37.8 v11.1,37.8 | U1.9 18.98,34.78 v19.15,34.95
  Bottom 0.152: v11.1,37.8 11.8,37.2 18.4,37.2 19.15,36.15 v19.15,34.95
POW_ON
  Top 0.152: R22.1 26.3,23.58 26.3,32.55 23.75,35.1 20.56,35.1 19.49,34.03 18.93,34.03 18.89,33.98 U1.7
RCVR_IN  (via drill 0.35)
  Top 0.152: v15,39.1 15,36.81 U1.19
  Bottom 0.152: Q2.C 15.58,42.25 R31.2 15.58,39.73 15,39.15 v15,39.1
SWDCLK
  Top 0.152: U1.25 12.4,36.15 12.4,38.25 11.5,39.15 10.27,39.15 TC1.4
SWDIO  (via drill 0.3)
  Top 0.152: U1.26 11.67,35.58 11.65,35.6 11.65,38 11.23,38.47 v11.2,38.5 | 10.36,40.43 10.31,40.48 | 10.36,40.43 10.82,40.43 v11.25,40 | TC1.2 10.36,40.43
  Bottom 0.152: v11.25,40 11.2,40 v11.2,38.5 11.2,38.45
VIN  (via drill 0.35, 0.5)
  Top 0.152: C19.2 C18.2 v27.1,12.1
  Top 0.254: C14.2 C15.2 33.15,31.22 U6.5 33.1,30.2 v32.35,30.2 | U4.5 27.11,14.31 C18.2 | U5.5 30.1,9.65 | 30.1,9.65 31.15,9.65 v31.2,9.7 | C30.2 30.6,11 C29.2 30.1,10.5 30.1,9.65
  Top 0.305: U2.1 45.19,16.33 JP1.1 47.85,16.28 47.85,14.25 45.8,12.2 R6.2 43.45,12.45 Q8.P$4
  Top 0.61: L1.1 v36.5,30.4
  Bottom 0.305: Q3.E 43.46,15.79 R9.2 44.7,15.97 R24.1 45.68,16.33 JP1.1 47.9,14.1 C7.1
  Bottom 0.61: v36.5,30.4 v36.5,29.5 37.5,28.5 R13.1 C20.1
  Bottom 1.016: R8.1 25.11,3.19 v26.2,2.1
  pour Route15 (isolate 0.254): 30.95,50.6 30.95,23.75 40.55,23.75 40.45,13.45 24.8,13.45 24.8,-0.45 50.75,-0.45 50.75,50.6
XMIT_DRV  (via drill 0.3)
  Top 0.152: v19.8,32.85 19.8,32.78 19.33,32.78 arc90 19.3,32.75 18.26,32.75 arc-90 U1.4 | R10.2 24.25,23.39 24.25,23.4 | 24.25,23.4 v24.25,23.45 | R12.2 23.93,23.08 24.25,23.4
  Bottom 0.152: v19.8,32.85 19.8,29 24.25,24.55 v24.25,23.45

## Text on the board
tNames: OT_BLE / Ver1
